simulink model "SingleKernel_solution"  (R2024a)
settings: Solver=VariableStepAuto  StartTime=0.0  StopTime=4096*4  RelTol=1e-3
PreLoadFcn:
  | load taps
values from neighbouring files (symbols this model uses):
  S = sum(round(C0))    [NormalizeCoef.m]
undefined symbols (not defined in the file or in its folder): amd, code, Evaluation, FIR_SingleStream, ipconfig, netlist, Platform, SingleStream, tmp, VCK190, Versal, vmctmp, vsva2197, xcvc1902
libraries: aieBasic x3, dspsrcs4 x1, dspobslib x1, vmcUtilities x1

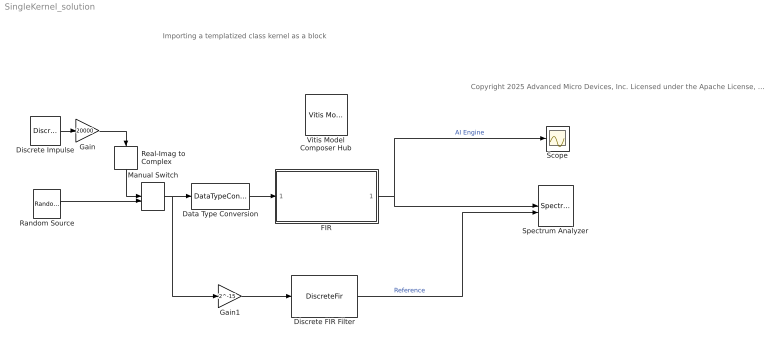
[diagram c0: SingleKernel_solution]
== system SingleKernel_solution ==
  note: Importing a templatized class kernel as a block
  note: Copyright 2025 Advanced Micro Devices, Inc. Licensed under the Apache License, Version 2.0 (the "License"); you may not use this file except in compliance with the License. You may obtain a copy of the License at http://www.apache.org/licenses/LICENSE-2.0 Unless required by applicable law or agreed to in writing, software distributed under the License is distributed on an "AS IS" BASIS, WITHOUT WARRANTIES OR CONDITIONS OF ANY KIND, either express or implied. See the License for the specific language governing permissions and limitations under the License.
  Data Type Conversion : DataTypeConversion  OutDataTypeStr=int16
  Discrete Impulse : dspsrcs4/Discrete  Impulse  Delay=0  SampleTime=1  FrameSample=512  OutputFrames=off  dataType=double  isSigned=on  wordLen=16  udDataType=sfix(16)  fracBitsMode=Best precision  numFracBits=15  OutDataTypeStr=double  LastOutDataTypeStr=double
  Discrete FIR Filter : DiscreteFir  Coefficients=taps'  InputProcessing=Columns as channels (frame based)
  FIR : Subsystem
  Gain : Gain  Gain=20000
  Gain1 : Gain  Gain=2^-15
  Manual Switch : ManualSwitch  CurrentSetting=0
  Random Source : dspobslib/Random Source  SrcType=Uniform  NormMethod=Ziggurat  CltLength=12  MinVal=-20000  MaxVal=20000  MeanVal=0  VarVal=1  RepMode=Not repeatable  rawSeed=1  IsInherit=off  SampMode=Discrete  SampTime=1  SampFrame=512  DataType=Double  OutComplex=Complex  OutputFrames=off
  Real-Imag to Complex : RealImagToComplex  Input=Real
  Scope : Scope
  Spectrum Analyzer : SpectrumAnalyzer  NumInputPorts=2  WindowPosition=[683.000000,125.000000,836.000000,436.000000,]  ScopeFrameLocation=window  Method=Welch  SampleRate=1  Span=1  StartFrequency=-0.5  StopFrequency=0.5  AveragingMethod=Running  YLimits=[-19.649799,105.80437418]  ShowLegend=on  AllowFFTLengthLessThanSamplesPerUpdate=on
  Vitis Model Composer Hub : vmcUtilities/Vitis Model Composer Hub  Tag=genX  CodeGeneration=off  SubsystemName=FIR  SubsystemType=AIENode  StartColumn=1  NumberOfColumns=1  TargetDirectory=./code  exportDesign=off  analyzeDesign=on  validateDesignOnHw=off  ExportType=AI Engines  IpVendor=xilinx.com  IpLibrary=hls  IpVersion=1.0  IpHWLanguage=Verilog  AieCompilerOptions={}  AieSimulatorOptions={}  CreateTestbench=on  TestbenchStackSize=10  RunRtlSim=off  RunCSim=off  RunAieSim=on  AieSimTimeout=50000  RunAieSimProfiling=off  LaunchVitisAnalyzer=off  PlotOutput=on  RunX86Sim=off  X86SimTimeout=10  GenHwImage=off  GenLibadfXo=off  GenHwValidationCode=off  PlatformType=Specify Platform  Platform=/opt/amd/Vitis/2024.2/base_platforms/xilinx_vck190_base_202420_1/xilinx_vck190_base_202420_1.xpfm  HwSystemType=Baremetal  HwValidationTarget=hw  ProjDevice=Versal VCK190 Evaluation Platform (xcvc1902-vsva2197-2MP-e-S)  ProjDevicePart=xcvc1902-vsva2197-2MP-e-S  AIEType=AIE  SamplePeriod=-1  ClockFrequency=200  DataPathParallelism=1  xilinxfamily=versalaicore  part=xcvc1902  speed=-2MP-e-S  package=vsva2197  directory=./netlist  testbench=off  incr_netlist=off  synthesis_tool=Vivado  clock_wrapper=Clock Enables  dbl_ovrd=According to Block Masks  dcm_input_clock_period=10  sysclk_period=10  simulink_period=1  eval_field=0  IPInfoJsonString="{\"DUTSubsystemName\":\"FIR\",\"AIESubsystem\":{\"SubsystemName\":\"FIR\",\"TargetDirectory\":\"./code\",\"AIEArrayConfig\":\"Use entire AIE array\",\"StartColumn\":\"0\",\"NumberOfColumns\":\"1\"},\"SubsystemTag\":\"AIENode\"}"  LogFileName=/home/amd/training/Import_AIE_class_kernel/completed/code/model_composer.log  NThreads=4  IPConfigFile=/tmp/vmctmp-amd/7036/ipconfig.json
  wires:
  Data Type Conversion/1 -> FIR/1(In1)
  FIR/1(Out1) -> Scope/1, Spectrum Analyzer/1  "AI Engine"
  Manual Switch/1 -> Gain1/1, Data Type Conversion/1
  Random Source/1 -> Manual Switch/2
  Discrete Impulse/1 -> Gain/1
  Real-Imag to Complex/1 -> Manual Switch/1
  Gain/1 -> Real-Imag to Complex/1
  Discrete FIR Filter/1 -> Spectrum Analyzer/2  "Reference"
  Gain1/1 -> Discrete FIR Filter/1

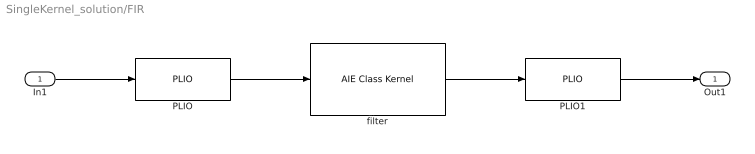
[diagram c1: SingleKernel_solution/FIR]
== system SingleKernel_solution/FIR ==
  In1 : Inport
  PLIO : aieBasic/PLIO  PlioWidth=64  PlioFreqSpec=off  PlioFreq=250  ColLocation=0  channel=0  blockJsonConstraints=[]  deprecateConstraints=0
  PLIO1 : aieBasic/PLIO  PlioWidth=64  PlioFreqSpec=off  PlioFreq=250  ColLocation=0  channel=0  blockJsonConstraints=[]  deprecateConstraints=0
  filter : aieBasic/AIE Class Kernel  KernelAllAttrs=s[12;12;9;9;19;14;21;23;21;23;24;21;15;17;12;24;26;26;26;27;28;9;21;23;23;23;24;25;14;19;19;29]@FunctionNameDeclFileNamePortNamesPortTypesPortSerializedTypesPortDirectionsPortWindowSizeEnablesPortWindowMarginEnablesPortBufferSizeEnablesPortBufferMarginEnablesPortSynchronicityEnablesPortSignalSizeEnablesPortBufferSizesPortBufferMarginsFunctionDeclFunctionTemplateSpecKindFunctionTemplateParamNamesFu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  PortNames={'sin'; 'sout'}  PortSerializedTypes={'{P{Tinput_stream{1{t{Scint16}}}}}'; '{P{Toutput_stream{1{t{Scint16}}}}}'}  PortWindowSizes={0.000000000000000000e+00; 0.000000000000000000e+00}  PortWindowMargins={0.000000000000000000e+00; 0.000000000000000000e+00}  PortSynchronicities={'auto', 'auto'}  PortSignalSizes={0.000000000000000000e+00; 5.120000000000000000e+02}  ClassTemplateSpecKind=implicit  ClassTemplateParamNames={'NSamples'; 'ShiftAcc'}  ClassTemplateParamKinds={'nontype'; 'nontype'}  ClassTemplateParamTypes={'int'; 'int'}  ClassTemplateParamValues={'512', '15'}  ClassCtorParamNames={'taps'}  ClassCtorParamSerializedTypes={'{R{Q1{C{Scint16}32}}}'}  ClassCtorParamValues={'[-82-253i;0-204i;11-35i;-198+273i;-642+467i;-1026+333i;-927;-226-73i;643+467i;984+1355i;550+1691i;0+647i;538-1656i;2860-3936i;6313-4587i;9113-2961i;9582;7421+2411i;3936+2860i;1023+1409i;-200-615i;0-1778i;517-1592i;467-643i;-192+140i;-882+287i;-1079;-755-245i;-273-198i;22+30i;63+194i;0+266i]'}  ClassIndex=1  ClassCtorIndex=1  ClassTabVisible=on  ClassTemplateParamsVisible=on  ClassCtorDeclVisible=on  ClassCtorParamsVisible=on  FunctionTabVisible=on  FunctionDecl=|  PortAttrs={ 'input', 'sin', 'input_stream_cint16 *', '', '', '', ''; 'output', 'sout', 'output_stream_cint16 *', '', '', '', '512' }  PortAttrsEnables={'off', 'off', 'off', 'off', 'off', 'off', 'off';'off', 'off', 'off', 'off', 'off', 'off', 'on'}  SampleTime=-1  ClassDeclTypeOptions=|  ClassDecl=|  ClassTemplateParams={ 'NSamples', 'int', '512'; 'ShiftAcc', 'int', '15' }  ClassTemplateParamsEnables={'off', 'off', 'on';'off', 'off', 'on'}  ClassCtorDeclTypeOptions=C[1 1]@t48@FIR_SingleStream(cint16 const ( & taps ) [ 32 ])  ClassCtorDecl=FIR_SingleStream(cint16 const ( & taps ) [ 32 ])  ClassCtorParams={ 'taps', 'cint16 const ( &) [ 32 ]', 'taps' }  KernelHeaderFile=src/aie_kernels/FirSingleStream.h  KernelClassName=SingleStream::FIR_SingleStream  KernelFunction=filter  KernelSourceFile=src/aie_kernels/FirSingleStream.cpp  KernelSearchPaths={}  PreProcOptions={}  blockJsonConstraints=[]
      | namespace SingleStream {
      | template < int NSamples, int ShiftAcc > 
      | void FIR_SingleStream::
      | filter(input_stream_cint16 * sin, output_stream_cint16 * sout);
      | }
      | C[1 1]@t90@namespace SingleStream {
      | template < int NSamples, int ShiftAcc > class FIR_SingleStream;
      | }
      | namespace SingleStream {
      | template < int NSamples, int ShiftAcc > class FIR_SingleStream;
      | }
  Out1 : Outport
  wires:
  In1/1 -> PLIO/1
  PLIO/1 -> filter/1
  PLIO1/1 -> Out1/1
  filter/1 -> PLIO1/1
